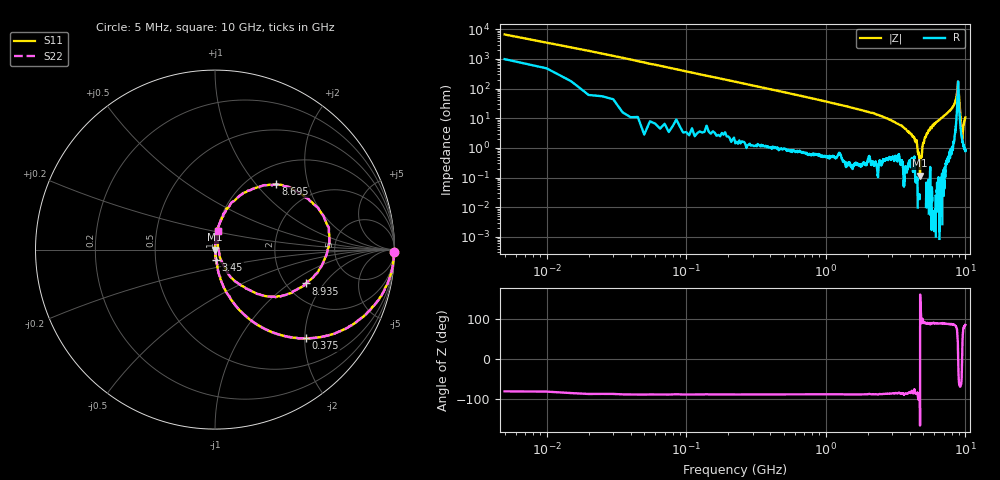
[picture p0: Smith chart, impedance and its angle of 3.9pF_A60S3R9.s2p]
! Amotech Co.,Ltd.
! http://www.amotech.co.kr/
! Part Number: A60S3R9
! These Parameters are Measured in Series Mode Connection
! Operation Temp=25[degC], DC Bias Voltage=0[V]
! Freq. Start=5[MHz] Stop=10[GHz], 2000[Steps]
! Date: Monday, July 13, 2020, 01:53:47
# GHZ S RI R 50.000000
!Freq.(Hz) S11(Real) S11(Imag) S21(Real) S21(Imag) S12(Real) S12(Imag) S22(Real) S22(Imag)
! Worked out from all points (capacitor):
!   2000 points, 5 MHz to 10 GHz, reference 50 ohm
!   read as one part in series: C = 4.19 pF near 55 MHz
!   lowest |Z| = 115 mohm at 4.73 GHz (marker M1)
!   series resonance near 4.737 GHz, so ESL is about 270 pH
!   S11 on the Smith chart (normalised r, x): 5 MHz: open; 375 MHz: 1.02, -2.03; 3.45 GHz: 1.01, -0.11; 8.695 GHz: 1.33, +1.28; 8.935 GHz: 2.53, -1.35; 10 GHz: 1.02, +0.21
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0.005  0.9976 -0.0148  0.00242 0.0148  0.00242 0.0148  0.9976 -0.0148
0.07  0.965 -0.178  0.035 0.178  0.035 0.178  0.965 -0.178
0.12  0.9065 -0.2861  0.0935 0.2861  0.0935 0.2861  0.9065 -0.2861
0.375  0.5072 -0.4944  0.4928 0.4944  0.4928 0.4944  0.5072 -0.4944
0.82  0.1743 -0.3724  0.8257 0.3724  0.8257 0.3724  0.1743 -0.3724
1.675  0.0428 -0.1953  0.9572 0.1953  0.9572 0.1953  0.0428 -0.1953
3.34  0.00981 -0.0604  0.9902 0.0604  0.9902 0.0604  0.00981 -0.0604
3.45  0.00659 -0.0569  0.9934 0.0569  0.9934 0.0569  0.00659 -0.0569
4.455  0.00111 -0.0178  0.9989 0.0178  0.9989 0.0178  0.00111 -0.0178
4.64  -0.000981 -0.00574  1.001 0.00574  1.001 0.00574  -0.000981 -0.00574
4.73  -0.00113 -0.000249  1.001 0.000249  1.001 0.000249  -0.00113 -0.000249
5.005  -0.000499 0.0147  1 -0.0147  1 -0.0147  -0.000499 0.0147
5.64  0.00252 0.0505  0.9975 -0.0505  0.9975 -0.0505  0.00252 0.0505
6.67  0.00934 0.0959  0.9907 -0.0959  0.9907 -0.0959  0.00934 0.0959
8.335  0.097 0.2662  0.903 -0.2662  0.903 -0.2662  0.097 0.2662
8.695  0.3406 0.3635  0.6594 -0.3635  0.6594 -0.3635  0.3406 0.3635
8.845  0.6347 0.1207  0.3653 -0.1207  0.3653 -0.1207  0.6347 0.1207
8.935  0.5058 -0.1887  0.4942 0.1887  0.4942 0.1887  0.5058 -0.1887
9.135  0.1085 -0.1737  0.8915 0.1737  0.8915 0.1737  0.1085 -0.1737
9.48  0.0186 0.00152  0.9814 -0.00152  0.9814 -0.00152  0.0186 0.00152
9.705  0.0149 0.0546  0.9851 -0.0546  0.9851 -0.0546  0.0149 0.0546
10  0.0188 0.1039  0.9812 -0.1039  0.9812 -0.1039  0.0188 0.1039
